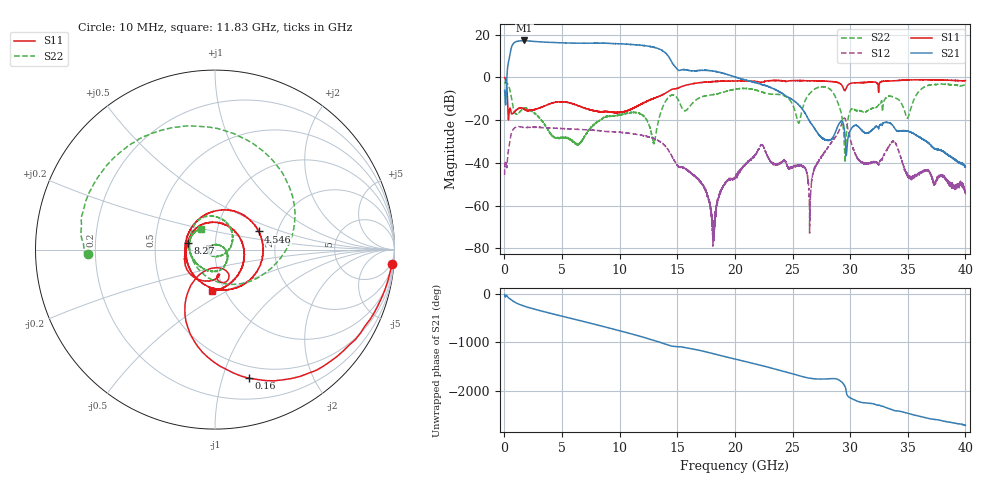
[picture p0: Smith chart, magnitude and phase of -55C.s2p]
!Agilent Technologies,E8363C,MY49030334,A.09.42.15
!Agilent E8363C: A.09.42.15
!Date: Thursday, February 26, 2026 09:27:15
!Correction: S11(Full 2 Port(1,2))
!S21(Full 2 Port(1,2))
!S12(Full 2 Port(1,2))
!S22(Full 2 Port(1,2))
!S2P File: Measurements: S11, S21, S12, S22:
# Hz S  dB  R 50
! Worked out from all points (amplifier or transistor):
!   6401 points, 10 MHz to 40 GHz, reference 50 ohm
!   highest |S21| = 17.2 dB at 1.71 GHz (marker M1)
!   |S21| within 3 dB of that: 614.9 MHz to 12.79 GHz (12.18 GHz wide, 182 % of centre)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
!   unconditionally stable (mu >= 1): start of sweep to end of sweep
!   at 6.671 GHz: K = 1.47, MAG = 16.1 dB, |S12| = -24.4 dB
!   at 20 GHz: K = 24.86, MAG = 6.4 dB, |S12| = -46.6 dB
!   at 40 GHz: K = 5653.55, MAG = -34.3 dB, |S12| = -54.5 dB
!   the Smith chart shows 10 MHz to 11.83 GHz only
!   S11 on the Smith chart (normalised r, x): 10 MHz: 3, -24; 160 MHz: 0.38, -1.23; 4.546 GHz: 1.60, +0.35; 8.27 GHz: 0.74, +0.06; 11.83 GHz: 0.87, -0.43
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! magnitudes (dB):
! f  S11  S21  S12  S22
! 10 MHz  -0.1  -6.1  -45.7  -3.0
! 160 MHz  -2.6  -5.9  -41.3  -2.4
! 691.1 MHz  -17.0  15.1  -25.0  -12.2
! 1.71 GHz  -14.9  17.2  -23.5  -14.4
! 4.546 GHz  -11.6  16.2  -23.8  -28.5
! 6.677 GHz  -13.9  15.9  -24.5  -30.0
! 8.27 GHz  -16.2  15.9  -25.0  -20.1
! 11.83 GHz  -12.6  15.0  -27.1  -17.2
! 13.34 GHz  -9.0  13.4  -29.6  -20.7
! 17.17 GHz  -2.4  3.2  -50.4  -9.1
! 18.12 GHz  -2.0  2.9  -69.9  -8.1
! 20 GHz  -1.7  0.1  -46.6  -5.6
! 22.33 GHz  -2.4  -3.4  -31.6  -6.8
! 25.52 GHz  -1.5  -12.8  -41.1  -21.4
! 26.67 GHz  -1.6  -22.1  -48.1  -6.6
! 28.47 GHz  -2.1  -28.4  -29.7  -6.8
! 29.46 GHz  -5.8  -23.0  -19.2  -27.6
! 31 GHz  -2.5  -24.8  -39.7  -15.9
! 33.34 GHz  -1.7  -21.2  -32.5  -8.8
! 34.98 GHz  -1.2  -25.1  -45.9  -19.1
! 36.48 GHz  -1.2  -29.5  -43.8  -4.5
! 40 GHz  -1.6  -42.0  -54.5  -3.5
